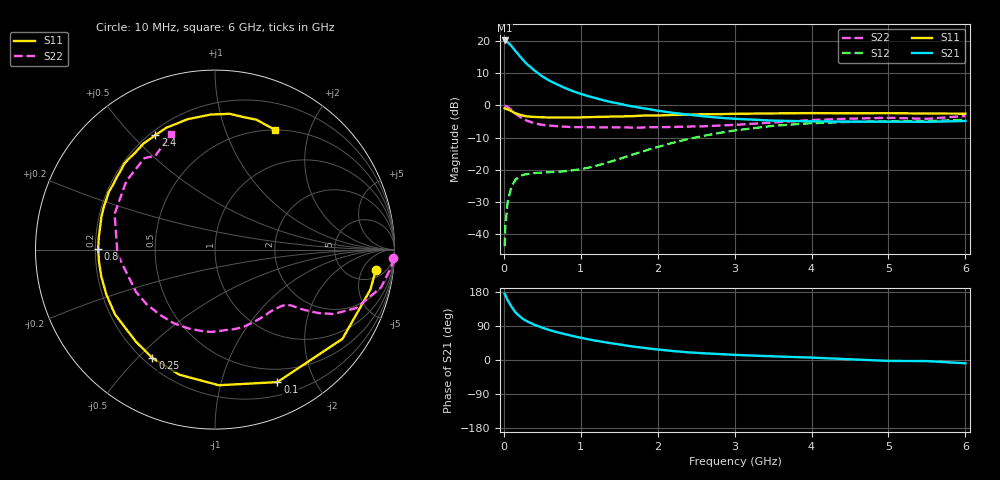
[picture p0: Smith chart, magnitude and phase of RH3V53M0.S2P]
! SIEMENS Small Signal Semiconductors
! BFR106
! Si NPN RF Bipolar Junction Transistor in SOT23
! VCE = 3.5 V  IC = 3 mA
! Common Emitter S-Parameters:  August  1996
# GHz  S  MA  R  50
!  f  S11  S21  S12  S22
! GHz  MAG  ANG  MAG  ANG  MAG  ANG  MAG  ANG
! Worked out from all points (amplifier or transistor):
!   36 points, 10 MHz to 6 GHz, reference 50 ohm
!   highest |S21| = 20.2 dB at 10 MHz (marker M1)
!   |S21| within 3 dB of that: start of sweep to 141.4 MHz
!   unconditionally stable (mu >= 1): 717.5 MHz to 2.016 GHz; 4.184 GHz to end of sweep
!   at 250 MHz: K = 0.39, MSG = 17.8 dB, |S12| = -21.6 dB
!   at 1.4 GHz: K = 1.21, MAG = 6.4 dB, |S12| = -17.4 dB
!   at 6 GHz: K = 1.02, MAG = -1.1 dB, |S12| = -4.5 dB
!   S11 on the Smith chart (normalised r, x): 10 MHz: 8, -10; 100 MHz: 0.34, -1.52; 250 MHz: 0.24, -0.55; 800 MHz: 0.21, +0.00; 2.4 GHz: 0.22, +0.58; 6 GHz: 0.50, +1.50
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0.01  0.903 -7.4  10.26 174.7  0.0065 86.9  0.9955 -2.8
0.02  0.8941 -14.4  10.21 171.1  0.0133 84.4  0.988 -5.4
0.05  0.867 -35.0  9.637 157.7  0.032 71.4  0.9482 -12.9
0.1  0.8159 -64.8  8.373 140.5  0.0554 57.4  0.851 -22.5
0.15  0.756 -88.4  7.047 126.0  0.0699 46.7  0.7518 -28.5
0.2  0.7248 -105.9  5.985 116.5  0.0781 40.5  0.6772 -31.5
0.25  0.6974 -120.0  5.089 108.2  0.0835 36.0  0.6185 -33.4
0.3  0.6763 -130.6  4.41 102.3  0.0858 33.7  0.5807 -34.7
0.4  0.6639 -147.0  3.482 92.9  0.089 31.0  0.5275 -36.2
0.5  0.6552 -157.5  2.831 85.2  0.0905 31.1  0.5006 -37.9
0.6  0.651 -166.8  2.412 78.6  0.0918 32.5  0.4859 -40.3
0.8  0.6511 179.7  1.858 68.0  0.0951 38.2  0.4671 -46.1
1.1  0.6591 163.6  1.394 54.6  0.1081 50.2  0.4588 -56.8
1.3  0.6664 155.4  1.203 47.4  0.1249 56.9  0.4568 -64.8
1.6  0.6794 143.9  1.001 37.8  0.1613 63.1  0.4555 -78.1
2.2  0.7125 124.0  0.768 23.6  0.2632 62.4  0.4634 -107.8
2.4  0.7187 117.6  0.72 20.2  0.3016 59.7  0.4706 -119.3
3.5  0.753 91.7  0.582 9.7  0.4824 37.0  0.5438 -177.2
4.5  0.7551 77.3  0.561 1.9  0.5541 16.3  0.624 142.4
5  0.7595 72.2  0.561 -2.4  0.5667 8.3  0.6438 127.7
5.5  0.7492 66.9  0.557 -2.9  0.5729 4.4  0.6196 122.4
6  0.7465 63.3  0.574 -8.7  0.5975 -3.5  0.6872 111.0
